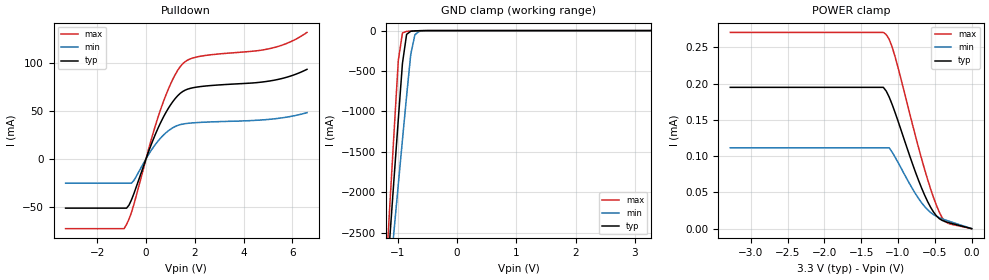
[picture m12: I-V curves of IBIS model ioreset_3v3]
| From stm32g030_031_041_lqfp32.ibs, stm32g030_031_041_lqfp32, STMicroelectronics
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|   Model ioreset_3v3
[Model]  ioreset_3v3
Model_type I/O_open_drain
Polarity   Inverting
Enable   Active-High
Vinl =   0.990000V
Vinh =   2.310000V
Vmeas =  1.650000V
Cref =   100.000000nF
Rref =   1.000000k
Vref =   3.300000V
C_comp   0.541680pF   0.532160pF   0.622160pF
[Temperature Range]   25.000000   0.125000k   -40.000000
[Pullup Reference]   3.300000V   2.700000V   3.600000V
[Pulldown Reference]   0.0V   0.0V   0.0V
[POWER Clamp Reference]   3.300000V   2.700000V   3.600000V
[GND Clamp Reference]   0.0V   0.0V   0.0V
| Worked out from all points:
|   slope of the pulldown table from 0 to 0.495 V, typ, clamps not added: 15.4 ohm
|   GND clamp passes 1 mA (typ) near -0.59 V on its own axis
[Pulldown]
|Voltage   I(typ)   I(min)   I(max)
-3.3V     -51.52mA   -25.42mA   -72.94mA
-900mV    -51.52mA   -25.42mA   -72.94mA
-700mV    -48.35mA   -25.42mA   -62.92mA
-500mV    -36.41mA   -22.69mA   -47.62mA
200mV     14.11mA    8.399mA    18.97mA
700mV     43.05mA    24.46mA    58.97mA
1.2V      63.12mA    33.85mA    88.19mA
1.6V      71.68mA    36.7mA     101.4mA
2.3V      75.66mA    38.14mA    107.4mA
5.2V      81.86mA    41.6mA     115.9mA
5.9V      86.24mA    44.14mA    122mA
6.6V      93.48mA    48.19mA    132mA
[GND_clamp]
|Voltage   I(typ)   I(min)   I(max)
-3.3V     -9.812A    -9.988A    -9.329A
-1.2V     -3.251A    -3.583A    -3.017A
-1.13V    -2.528A    -3.02A     -2.122A
-1.06V    -1.808A    -2.459A    -1.234A
-990mV    -1.097A    -1.901A    -369.4mA
-920mV    -404.3mA   -1.349A    -29.79mA
-850mV    -46.63mA   -808.1mA   -9.867mA
-780mV    -8.596mA   -293.7mA   -6.34mA
-710mV    -3.483mA   -50.92mA   -3.779mA
-640mV    -1.689mA   -10.39mA   -1.818mA
-430mV    -117.5uA   -209uA     -95.53uA
3.28V     0A         0A         0A
[POWER_clamp]
|Voltage   I(typ)   I(min)   I(max)
-3.28V    194.9uA    111.5uA    270.7uA
-1.2V     194.9uA    111.5uA    270.7uA
-1.16V    189.6uA    111.5uA    267.5uA
-1.12V    181.3uA    111.5uA    260.9uA
-1.04V    159.9uA    98.51uA    236.9uA
-800mV    88.19uA    54.24uA    142uA
-680mV    55.9uA     35.7uA     96.15uA
-560mV    29.86uA    22.47uA    55.4uA
-440mV    13.83uA    15.14uA    22.69uA
-400mV    11.32uA    13.54uA    14.87uA
-320mV    8.512uA    10.71uA    7.327uA
0V        0A         0A         0A
[Ramp]
| variable   typ   min   max
dV/dt_r  1.97933/62.68895n   1.61903/54.83523n   2.15945/66.91529n
dV/dt_f  1.97933/5.65840n   1.61903/9.16002n   2.15945/4.39127n
R_load = 40.000000k
